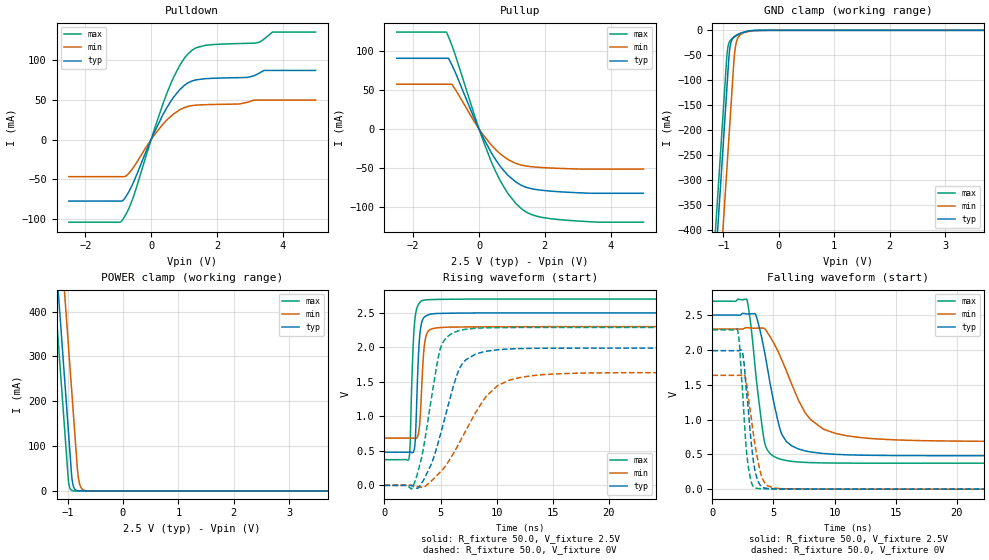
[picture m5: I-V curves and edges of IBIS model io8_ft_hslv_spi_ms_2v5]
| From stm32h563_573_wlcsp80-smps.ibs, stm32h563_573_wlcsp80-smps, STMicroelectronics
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[Model]   io8_ft_hslv_spi_ms_2v5
Model_type I/O
Polarity   Non-Inverting
Enable   Active-Low
| CAP_THRESHOLD on pad IOFT is "UDTCAPC" :
| Rising=20.0% of vddiom   Falling=80.0% of vddiom
| C_comp min and max val. don't necessarily correlate with the min and max pvt
| but are the smallest and greatest pad capacitance found.
| var   typ   min   max
C_comp   4.85183pF  4.77592pF  4.93407pF
|C_comp_pullup   3.10520pF  2.91265pF  2.94055pF
|C_comp_pulldown   1.74663pF  1.86327pF  1.99352pF
Vinl = 690.0mV
Vinh = 1.89V
Vmeas = 1.25V   | Reference voltage for timing measurements
Cref  = 50.0pF   | Timing specification test load capacitance value
Rref  = 100.0MOhm   | Timing specification test load resistance value
Vref  = 1.25V   | Timing specification test load voltage
[Model Spec]
| TIME_THRESHOLD on pin ZIV11 is "CMOS" :
| Rising=40.0% of vdd   Falling=60.0% of vdd
Vinl 989.80000mV 917.80000mV 1.06580V
Vinh 1.40320V 1.29620V 1.49120V
| variable   typ   min   max
[Temperature Range] 25.0 125.0 -40.0
| variable   typ   min   max
[Voltage Range] 2.5V 2.3V 2.7V
| variable   typ   min   max
[POWER Clamp Reference] 2.5V 2.3V 2.7V
| variable   typ   min   max
[GND Clamp Reference] 0V 0V 0V
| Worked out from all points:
|   slope of the pulldown table from 0 to 0.375 V, typ, clamps not added: 11.5 ohm
|   slope of the pullup table from 0 to 0.375 V, typ, clamps not added: 12.3 ohm
|   GND clamp passes 1 mA (typ) near -0.52 V on its own axis
|   POWER clamp passes 1 mA (typ) near -0.84 V on its own axis
|   rising waveform, R_fixture 50.0, V_fixture 2.5V: 20-80 % time 297ps typ, 334ps min, 298ps max; typ from 0.481 V to 2.5 V
|   falling waveform, R_fixture 50.0, V_fixture 2.5V: 20-80 % time 1.37ns typ, 2.63ns min, 888ps max; typ from 2.5 V to 0.481 V
|   rising waveform, R_fixture 50.0, V_fixture 0V: 20-80 % time 2.07ns typ, 3.54ns min, 1.39ns max; typ from 0 V to 1.99 V
|   falling waveform, R_fixture 50.0, V_fixture 0V: 20-80 % time 662ps typ, 864ps min, 533ps max; typ from 1.99 V to 0 V
[POWER Clamp]
-2.5V     2.708A     2.899A     2.597A
-1.23V    548.8mA    740.2mA    437.5mA
-1.16V    429.8mA    621.2mA    318.5mA
-1.07V    276.8mA    468.2mA    165.5mA
-1.03V    208.8mA    400.2mA    97.53mA
-980mV    123.8mA    315.2mA    17.95mA
-920mV    26.3mA     213.2mA    906uA
-880mV    5.543mA    145.2mA    123.7uA
-810mV    363.5uA    33.6mA     3.797uA
-770mV    76.62uA    10.47mA    518.9nA
-700mV    5.026uA    1.361mA    16.14nA
5V        0A         0A         0A
[GND Clamp]
-2.5V     -2.771A    -2.933A    -2.706A
-1.21V    -578.3mA   -739.7mA   -512.8mA
-950mV    -136.3mA   -297.7mA   -70.75mA
-930mV    -102.3mA   -263.7mA   -41.56mA
-900mV    -51.97mA   -212.7mA   -25.14mA
-880mV    -32.59mA   -178.7mA   -20.84mA
-850mV    -19.78mA   -127.7mA   -17.15mA
-810mV    -13.22mA   -60.17mA   -13.75mA
-780mV    -10.64mA   -30.96mA   -11.62mA
-730mV    -7.637mA   -13.21mA   -8.533mA
-430mV    -217.7uA   -562.2uA   -113.2uA
5V        7.27nA     1.305uA    342.4pA
| variable   typ   min   max
[Pullup Reference] 2.5V 2.3V 2.7V
| variable   typ   min   max
[Pulldown Reference] 0V 0V 0V
[Pullup]
-2.5V     90.56mA    57.35mA    124.1mA
-990mV    90.56mA    57.35mA    124.1mA
-930mV    90.56mA    57.35mA    118.3mA
-830mV    82.36mA    57.35mA    107.7mA
0V        12.15pA    815pA      8.64pA
350mV     -28.74mA   -19.44mA   -39.66mA
610mV     -45.85mA   -30.67mA   -63.5mA
870mV     -59.1mA    -39.02mA   -82.25mA
1.29V     -72.3mA    -46.39mA   -102.3mA
1.7V      -77.4mA    -48.84mA   -111.2mA
2.27V     -80.02mA   -50.27mA   -115.5mA
5V        -82.5mA    -51.48mA   -119.5mA
[Pulldown]
-2.5V     -77.63mA   -46.84mA   -104.3mA
-870mV    -77.25mA   -46.84mA   -101.4mA
-550mV    -55.3mA    -35.88mA   -73.72mA
90mV      8.401mA    5.299mA    11.79mA
610mV     49.03mA    29.76mA    71.69mA
870mV     62.92mA    37.48mA    93.62mA
1.23V     73.63mA    42.72mA    112.2mA
1.64V     76.78mA    44.01mA    118.8mA
2.94V     78.48mA    47.15mA    121.4mA
3.24V     82.82mA    49.81mA    122.4mA
3.69V     87.21mA    49.81mA    135.6mA
5V        87.21mA    49.81mA    135.6mA
[Ramp]
dV/dt_r 1.19347V/2.0633ns 980.80932mV/3.52276ns 1.37307V/1.38972ns
dV/dt_f 1.21165V/1.36946ns 969.2603mV/2.61944ns 1.39628V/887.31972ps
R_load = 50.0
| Removed startup time: 0s 0s 0s  .
| Removed end time: 34.4ns.
[Rising Waveform]
R_fixture   = 50.0
V_fixture   = 2.5V
V_fixture_min = 2.3V
V_fixture_max = 2.7V
0s        480.6mV    684.6mV    372.9mV
2.2ns     480.8mV    684.6mV    394.4mV
2.3ns     480.9mV    684.7mV    637mV
2.65ns    513.7mV    680.5mV    2.286V
2.75ns    655.1mV    677.9mV    2.452V
3.1ns     2.078V     820.1mV    2.639V
3.35ns    2.375V     1.518V     2.677V
3.7ns     2.456V     2.161V     2.688V
4.55ns    2.49V      2.28V      2.694V
34.4ns    2.5V       2.3V       2.7V
| Removed startup time: 0s 0s 0s  .
| Removed end time: 49.4ns.
[Falling Waveform]
R_fixture   = 50.0
V_fixture   = 2.5V
V_fixture_min = 2.3V
V_fixture_max = 2.7V
0s        2.5V       2.3V       2.7V
2.8ns     2.517V     2.32V      2.73V
3.15ns    2.518V     2.314V     2.351V
3.55ns    2.506V     2.312V     1.66V
4.25ns    1.989V     2.308V     692mV
5.6ns     827.5mV    1.889V     429.2mV
6.5ns     620.9mV    1.504V     399.3mV
8.05ns    534.1mV    997.4mV    381.2mV
11.1ns    492.9mV    764.1mV    374.1mV
49.4ns    480.6mV    684.6mV    372.9mV
| Removed startup time: 0s 0s 0s  .
| Removed end time: 49.4ns.
[Rising Waveform]
R_fixture   = 50.0
V_fixture   = 0V
V_fixture_min = 0V
V_fixture_max = 0V
0s        101.5nV    479.1nV    83.46nV
2.5ns     -8.998mV   738.8uV    -31.99mV
3.4ns     53.47mV    -28.37mV   473.2mV
4.2ns     316.4mV    65.9mV     1.277V
5ns       743mV      196mV      1.989V
6.6ns     1.659V     593.8mV    2.24V
7.3ns     1.824V     807.7mV    2.263V
9.1ns     1.944V     1.295V     2.283V
13.1ns    1.985V     1.589V     2.288V
49.4ns    1.989V     1.635V     2.288V
| Removed startup time: 0s 0s 0s  .
| Removed end time: 24.4ns.
[Falling Waveform]
R_fixture   = 50.0
V_fixture   = 0V
V_fixture_min = 0V
V_fixture_max = 0V
0s        1.989V     1.635V     2.288V
2.05ns    1.989V     1.635V     2.29V
2.2ns     1.99V      1.635V     2.117V
2.45ns    1.973V     1.643V     1.469V
2.85ns    1.301V     1.455V     448.5mV
3.15ns    725.6mV    1.066V     128.2mV
3.45ns    299.7mV    683.2mV    22.42mV
4.1ns     27.9mV     152.8mV    5.865mV
5ns       5.987mV    16.11mV    3.063mV
24.4ns    1.938uV    19.59uV    322.6nV
